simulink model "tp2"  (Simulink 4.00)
settings: Solver=ode45  StartTime=0.0  StopTime=tfinal  RelTol=1e-3
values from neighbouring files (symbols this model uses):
  m = 4    [demo1dat.m]    (also in demo2dat.m = 3; essai1dat.m; essai2dat.m = 6; mynlcmpc.m = mp(1:max(size(mp))-1))
  model = tfd2step(1.6,delt,1,g)    [essai2dat.m]    (also in mynlcmpc.m = modelpd(:,1:nu); mynlcmpc2.m = modelpd(:,1:nu); mynlcmpc3.m = modelpd(:,1:nu); scrtp1.m = tfd2step(tfinal,Ts,1,g))
  p = 10    [demo1dat.m]    (also in demo2dat.m; essai1dat.m; essai2dat.m; mynlcmpc.m = mp(max(size(mp))))
  Ts = [tsamp 0]    [mynlcmpc.m]    (also in mynlcmpc2.m; mynlcmpc3.m; scrtp1.m = 0.1; Smpc.m)
  ulim = [-5 40 3]    [essai2dat.m]    (also in mynlcmpc.m = [-inf*ones(1,nu) inf*ones(1,nu) 1e6*ones(1,nu)]; mynlcmpc2.m = [-inf*ones(1,nu) inf*ones(1,nu) 1e6*ones(1,nu)]; mynlcmpc3.m = [-inf*ones(1,nu) inf*ones(1,nu) 1e6*ones(1,nu)]; pmlin.m = [-10*[1 1] 10*[1 1] 2*[1 1]])
  uwt = [0 0]    [demo1dat.m]    (also in demo2dat.m = 0.6*[1 1]; essai1dat.m; essai2dat.m = 1; mynlcmpc.m = ryuwt(:,2*ny+1:2*ny+nu))
  ylim = [-40 40]    [essai2dat.m]    (also in mynlcmpc.m = [ylim; ylim(N,:)]; mynlcmpc2.m = [ylim; ylim(N,:)]; mynlcmpc3.m = [ylim; ylim(N,:)]; pmlin.m = [])
  ywt = [1 1]    [demo1dat.m]    (also in demo2dat.m = [0.2,0,1]; essai1dat.m; essai2dat.m = 1; mynlcmpc.m = ryuwt(:,ny+1:2*ny))

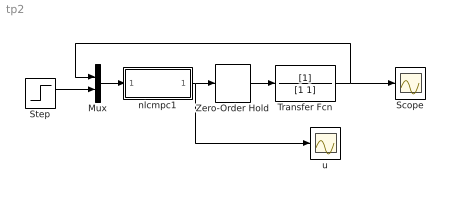
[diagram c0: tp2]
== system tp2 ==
  Mux : Mux  Inputs=2
  Scope : Scope
  Step : Step  Time=1  Before=0  After=1  SampleTime=0
  Transfer Fcn : TransferFcn  Numerator=[1]  Denominator=[1 1]  AbsoluteTolerance=auto  Realization=auto
  Zero-Order Hold : ZeroOrderHold  SampleTime=Ts
  nlcmpc1 : Subsystem  AncestorBlock=nlmpclib/nlcmpc  mask(myCMPC-SIMULINK){modelpd=[model []], yuwt=[ywt uwt], mp=[m p], yulim=[ylim ulim], tfilter=[], ud0=[0 []]}
      mask help: Masked MATLAB function block calls nlcmpc, links CMPC and SIMULINK.
  u : Scope
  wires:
  Zero-Order Hold/1 -> Transfer Fcn/1
  Transfer Fcn/1 -> Scope/1, Mux/1
  nlcmpc1/1(Out1) -> Zero-Order Hold/1, u/1
  Mux/1 -> nlcmpc1/1(In1)
  Step/1 -> Mux/2

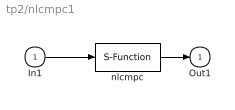
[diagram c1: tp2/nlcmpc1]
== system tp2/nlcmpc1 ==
  In1 : Inport  Port=1  LatchInput=off
  nlcmpc : S-Function  FunctionName=mynlcmpc3  Parameters=modelpd,mp,tfilter,yuwt,ud0,yulim  PortCounts=[]  SFunctionModules=''
  Out1 : Outport  Port=1  InitialOutput=0
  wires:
  In1/1 -> nlcmpc/1
  nlcmpc/1 -> Out1/1
